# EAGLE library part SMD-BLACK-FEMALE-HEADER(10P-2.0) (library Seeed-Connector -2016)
320030097
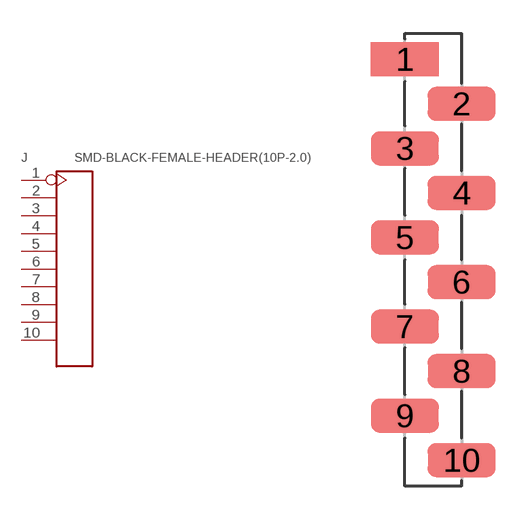
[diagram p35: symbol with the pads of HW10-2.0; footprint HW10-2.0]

Designator prefix J

## SMD-BLACK-FEMALE-HEADER(10P-2.0)-2-SMD (VALUE: 10P-SMD-2.0)  [HW10-2.0]
1  1
2  2
3  3
4  4
5  5
6  6
7  7
8  8
9  9
10  10

## Footprint HW10-2.0 (pad centres in mm)
smd 3.048 x 1.524: 1 -1.27,9; 2 1.27,7; 3 -1.27,5; 4 1.27,3; 5 -1.27,1; 6 1.27,-1; 7 -1.27,-3; 8 1.27,-5; 9 -1.27,-7; 10 1.27,-9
